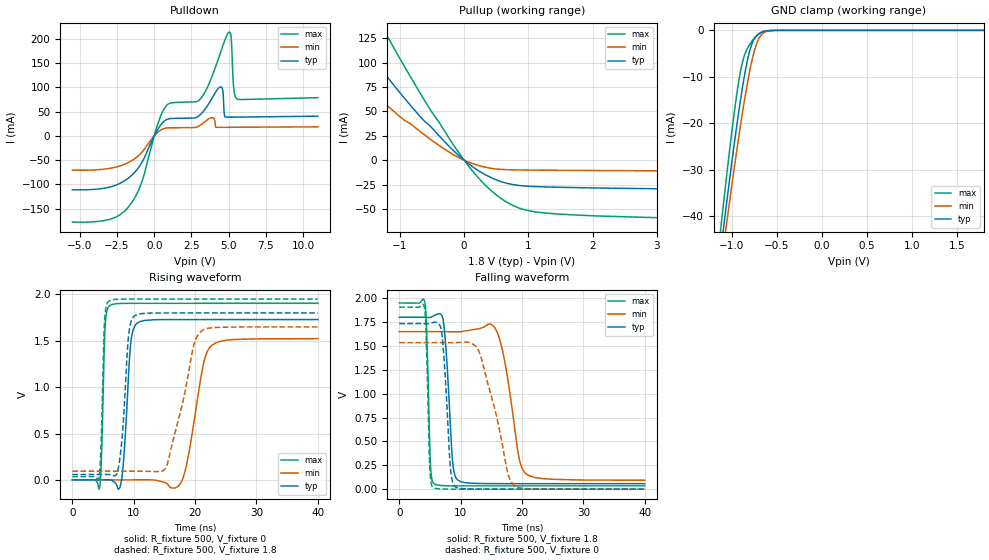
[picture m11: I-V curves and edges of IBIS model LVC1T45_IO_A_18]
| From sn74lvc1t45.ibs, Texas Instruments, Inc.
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[Model]   LVC1T45_IO_A_18
Model_type  I/O
Vinl=0.5775
Vinh=1.2675
Enable   Active-Low
Vref =   0
Rref =   2000
Cref =   15p
Vmeas =   0.9
| variable   typ   min   max
C_comp   7.41pF   6.57pF   8.25pF
| C_pullup   10.66pF   9.62pF   11.99pF
| C_pulldown   11.25pF   8.17pF   15.60pF
| C_tri-state   7.41pF   6.57pF   8.25pF
[Temperature Range]   40   100   -40
| Ambient temperature   25   85   -40
[Voltage range]   1.8   1.65   1.95
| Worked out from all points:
|   slope of the pulldown table from 0 to 0.27 V, typ, clamps not added: 17.9 ohm
|   slope of the pullup table from 0 to 0.27 V, typ, clamps not added: 21.3 ohm
|   GND clamp passes 1 mA (typ) near -0.71 V on its own axis
|   rising waveform, R_fixture 500, V_fixture 0: 20-80 % time 888ps typ, 2.24ns min, 441ps max; typ from 0 V to 1.73 V
|   falling waveform, R_fixture 500, V_fixture 1.8: 20-80 % time 921ps typ, 2.13ns min, 482ps max; typ from 1.8 V to 0.058 V
|   rising waveform, R_fixture 500, V_fixture 1.8: 20-80 % time 988ps typ, 3.09ns min, 458ps max; typ from 0.058 V to 1.8 V
|   falling waveform, R_fixture 500, V_fixture 0: 20-80 % time 923ps typ, 3.29ns min, 465ps max; typ from 1.73 V to 0 V
[GND Clamp]
| LVC1T45_IO_A_18
|   Voltage   I(typ)   I(min)   I(max)
-5.5V     -910.9mA   -836.3mA   -1.031A
-1.15V    -51.97mA   -55.4mA    -47.66mA
-1.115V   -46.31mA   -50.15mA   -41.36mA
-1.085V   -41.55mA   -45.71mA   -36.08mA
-1.07V    -39.19mA   -43.51mA   -33.49mA
-1.055V   -36.86mA   -41.33mA   -30.93mA
-960mV    -22.72mA   -27.97mA   -15.92mA
-880mV    -12.18mA   -17.61mA   -6.789mA
-775mV    -2.883mA   -6.453mA   -2.321mA
-710mV    -920.7uA   -2.212mA   -923.3uA
-650mV    -302.1uA   -584.3uA   -254.3uA
1.8V      6.037pA    540.4pA    4.293pA
[Pulldown]
| LVC1T45_IO_A_18
|   Voltage   I(typ)   I(min)   I(max)
-5.5V     -111.4mA   -70.76mA   -178.1mA
-1.725V   -86.91mA   -54.76mA   -146.6mA
655mV     29.91mA    15.28mA    55.28mA
3.135V    44.94mA    22.73mA    77.39mA
4.465V    101.2mA    17.68mA    172.9mA
4.615V    92.58mA    17.71mA    186.3mA
4.74V     40.47mA    17.73mA    197mA
5.03V     38.76mA    17.77mA    214.5mA
5.175V    38.77mA    17.8mA     201.9mA
5.36V     38.8mA     17.83mA    94.76mA
5.55V     38.84mA    17.86mA    76.62mA
11V       40.75mA    18.73mA    78.98mA
[Pullup]
| LVC1T45_IO_A_18
|   Voltage   I(typ)   I(min)   I(max)
-5.5V     441.6mA    75.79mA    604.5mA
-5.24V    422.8mA    99.59mA    579.6mA
-5.09V    411.7mA    138.7mA    565.1mA
-2.575V   205.3mA    144.6mA    291.7mA
-1.905V   146.3mA    100.5mA    211.7mA
-1.675V   126.2mA    85.63mA    184.2mA
-1.22V    87.44mA    57.45mA    130.1mA
-520mV    34.49mA    21.24mA    51.22mA
140mV     -7.072mA   -3.66mA    -11.83mA
575mV     -22mA      -9.421mA   -39.34mA
1.08V     -26.97mA   -10.16mA   -52.81mA
11V       -33.54mA   -12.74mA   -67.97mA
[Ramp]
| LVC1T45_IO_A_18
| variable   typ   min   max
dV/dt_r   1.10/9.51E-10   0.97/2.38E-09   1.20/4.72E-10
dV/dt_f   1.07/9.47E-10   0.98/2.28E-09   1.17/5.00E-10
R_load = 500
[Rising Waveform]
| LVC1T45_IO_A_18
R_fixture =   500
C_fixture =   0
L_fixture =   0
V_fixture =   0
V_fixture_min = 0
V_fixture_max = 0
|   Time   V(typ)   V(min)   V(max)
0s        136.8pV    359.1pV    79.4pV
4.41ns    -53.67uV   2.884uV    -90.84mV
5.31ns    1.267mV    -11.6uV    1.632V
6.095ns   655.8uV    1.823uV    1.88V
7.95ns    -24.45mV   -28.11uV   1.903V
9.475ns   1.456V     -64.19uV   1.904V
10.58ns   1.691V     748.7uV    1.904V
17.68ns   1.729V     -32.75mV   1.904V
22.81ns   1.729V     1.455V     1.904V
40ns      1.729V     1.523V     1.904V
[Falling Waveform]
| LVC1T45_IO_A_18
R_fixture =   500
C_fixture =   0
L_fixture =   0
V_fixture =   1.8
V_fixture_min = 1.65
V_fixture_max = 1.95
|   Time   V(typ)   V(min)   V(max)
0s        1.8V       1.65V      1.95V
4.165ns   1.8V       1.65V      1.959V
5.09ns    1.799V     1.65V      258.3mV
5.67ns    1.818V     1.65V      57.95mV
7.19ns    1.761V     1.65V      37.13mV
8.685ns   299.9mV    1.648V     35.03mV
9.575ns   93.56mV    1.647V     34.72mV
15.83ns   58.02mV    1.662V     34.49mV
20.72ns   57.67mV    158.4mV    34.49mV
40ns      57.62mV    93.41mV    34.48mV
[Rising Waveform]
| LVC1T45_IO_A_18
R_fixture =   500
C_fixture =   0
L_fixture =   0
V_fixture =   1.8
V_fixture_min = 1.65
V_fixture_max = 1.95
|   Time   V(typ)   V(min)   V(max)
0s        57.57mV    93.15mV    34.46mV
4.32ns    57.53mV    93.15mV    21.31mV
5.215ns   58.5mV     93.14mV    1.681V
5.92ns    57.72mV    93.15mV    1.927V
7.585ns   166mV      93.13mV    1.949V
9.13ns    1.542V     93.14mV    1.95V
10.12ns   1.77V      93.52mV    1.95V
15.29ns   1.8V       136.1mV    1.95V
21ns      1.8V       1.604V     1.95V
40ns      1.8V       1.65V      1.95V
[Falling Waveform]
| LVC1T45_IO_A_18
R_fixture =   500
C_fixture =   0
L_fixture =   0
V_fixture =   0
V_fixture_min = 0
V_fixture_max = 0
|   Time   V(typ)   V(min)   V(max)
0s        1.734V     1.535V     1.907V
4.115ns   1.734V     1.535V     1.897V
4.99ns    1.733V     1.535V     217.1mV
5.505ns   1.745V     1.535V     18.77mV
6.93ns    1.637V     1.535V     1.888mV
8.33ns    231.5mV    1.534V     382.3uV
9.13ns    25.07mV    1.535V     179.1uV
13.05ns   495.2uV    1.435V     33.65uV
18.75ns   74.26uV    38.01mV    27.03uV
40ns      42.23uV    102.9uV    17.43uV
